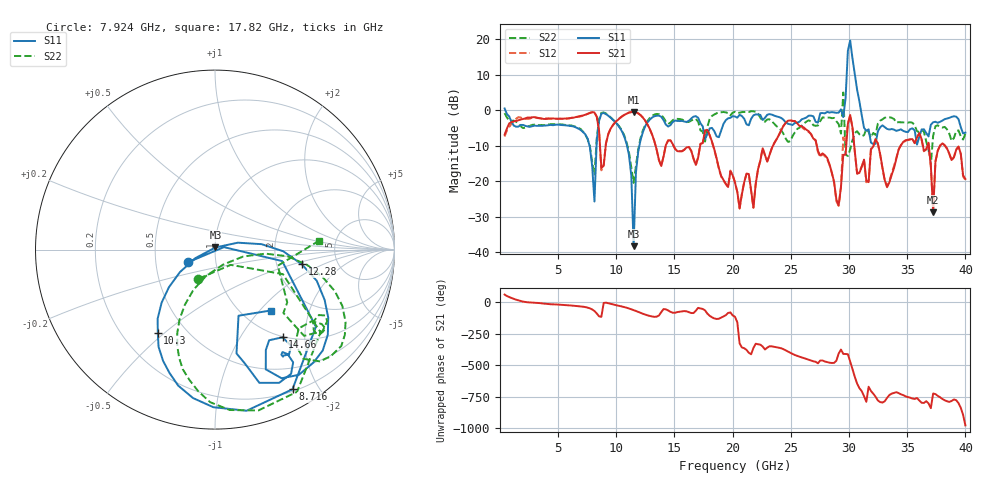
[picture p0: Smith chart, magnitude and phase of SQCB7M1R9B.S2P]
! Network Analyzer HP8722ES.07.66: Jul 25, 2000 Serial No. US39175408
! 26 Oct 2004  11:32:37
! Frequency  S11  S21  S12  S22
# HZ  S  DB R  50
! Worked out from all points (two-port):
!   201 points, 400 MHz to 40 GHz, reference 50 ohm
!   highest |S21| = -0.50 dB at 11.49 GHz (marker M1); lowest = -28.8 dB at 37.23 GHz (marker M2)
!   |S21| within 3 dB of the highest: 911.9 MHz to 8.404 GHz (7.492 GHz wide, 161 % of centre); 9.88 GHz to 12.58 GHz (2.704 GHz wide, 24.1 % of centre)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
!   lowest |S11| = -38.3 dB at 11.49 GHz (marker M3), VSWR 1.02, Z = 50.3 + j1.2 ohm
!   |S11| at or under -10 dB: 7.698 GHz to 8.302 GHz (604.2 MHz wide, 7.55 % of centre); 10.92 GHz to 11.98 GHz (1.064 GHz wide, 9.29 % of centre)
!   |S22| runs from -20.4 to 5.0 dB; largest |S21 - S12| = 0.19
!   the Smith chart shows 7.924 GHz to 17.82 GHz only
!   S11 on the Smith chart (normalised r, x): 7.924 GHz: 0.73, -0.11; 8.716 GHz: 0.22, -1.68; 10.3 GHz: 0.35, -0.48; 12.28 GHz: 2.78, -0.60; 14.66 GHz: 0.99, -1.56; 17.82 GHz: 1.33, -1.15
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4e8  0.49 -30.6  -6.88 60.7  -7.40 66.3  -0.81 -22.3
7.132e9  -6.11 -131.6  -1.48 -35.4  -1.57 -36.3  -6.03 -119.1
7.924e9  -15.64 -154.9  -0.57 -57.1  -0.55 -57.8  -14.56 -119.7
8.716e9  -1.01 -61.0  -16.27 -115.8  -16.92 -117.1  -0.77 -60.0
1.03e10  -4.97 -124.4  -2.25 -29.9  -2.21 -30.3  -4.78 -111.3
1.1488e10  -38.26 77.3  -0.50 -62.7  -0.47 -63.4  -20.45 -60.9
1.228e10  -6.19 -9.6  -2.09 -91.5  -2.04 -91.9  -5.71 -9.3
1.3666e10  -1.52 -56.2  -14.04 -105.3  -14.10 -104.8  -1.14 -42.7
1.4656e10  -4.20 -52.4  -8.49 -76.6  -8.49 -77.7  -3.47 -36.5
1.7824e10  -6.75 -47.6  -5.54 -90.5  -5.59 -91.8  -4.70 4.9
2.02e10  -1.78 -36.8  -20.41 -115.6  -20.25 -116.3  -0.45 -26.7
2.6932e10  -1.72 -58.2  -7.99 -108.6  -7.94 -108.3  -4.23 11.1
2.911e10  -0.69 -49.1  -26.77 -47.0  -26.92 -45.7  -3.92 -73.8
2.9506e10  -1.95 26.4  -12.57 -50.5  -7.65 -61.1  4.99 117.1
2.9704e10  3.38 -42.9  -12.51 -50.8  -9.44 -65.3  -12.47 -142.4
2.9902e10  16.77 -81.8  -3.81 -52.7  -3.80 -53.8  -12.91 -46.5
3.01e10  19.62 -132.1  -1.34 -111.0  -1.41 -111.3  -11.03 -50.6
3.0298e10  14.54 -164.1  -4.95 -172.7  -5.00 -174.9  -8.36 -62.6
3.0694e10  5.75 -26.6  -17.89 74.2  -17.81 69.9  -5.92 81.8
3.3466e10  -5.44 129.7  -20.33 -16.5  -19.99 -18.5  -2.01 141.6
3.7228e10  -3.38 -115.8  -28.75 -4.0  -27.63 0.7  -7.19 -44.8
4e10  -6.30 125.4  -19.35 102.3  -19.59 101.3  -6.63 -179.3
